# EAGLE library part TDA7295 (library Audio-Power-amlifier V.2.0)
The TDA7295 is a monolithic integrated circuit in Multiwatt15 package, intended for use as audio class AB amplifier in Hi-Fi field applications (Home Stereo, self powered loudspeakers, Topclass TV). Thanks to the wide voltage range and to the high out current capability it is able to supply the highest power into both 4W and 8W loads even in presence of poor supply regulation, with high Supply Voltage Rejection. The built in muting function with turn on delay simplifies the remote operation avoiding switching on-off noises.
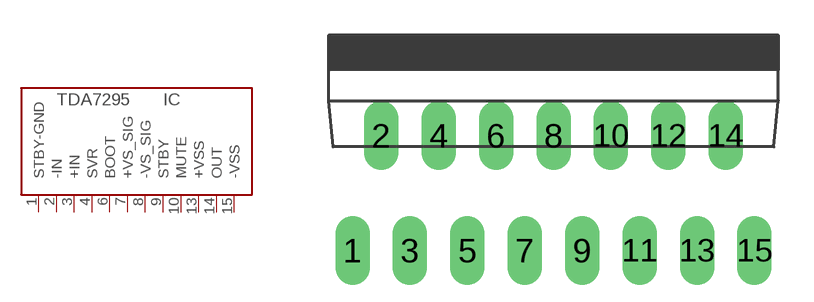
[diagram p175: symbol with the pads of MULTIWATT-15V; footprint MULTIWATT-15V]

Designator prefix IC

## TDA7295  [MULTIWATT-15V]
1  STBY-GND  in
2  -IN  in
3  +IN  in
4  SVR
6  BOOT
7  +VS_SIG  pwr
8  -VS_SIG  pwr
9  STBY  in
10  MUTE  in
13  +VSS  pwr
14  OUT  out
15  -VSS  pwr

## Footprint MULTIWATT-15V (pad centres in mm)
Multiwatt 15 vertical
drill 1.016 long: 1 -8.89,-5.08; 2 -7.62,0; 3 -6.35,-5.08; 4 -5.08,0; 5 -3.81,-5.08; 6 -2.54,0; 7 -1.27,-5.08; 8 0,0; 9 1.27,-5.08; 10 2.54,0; 11 3.81,-5.08; 12 5.08,0; 13 6.35,-5.08; 14 7.62,0; 15 8.89,-5.08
